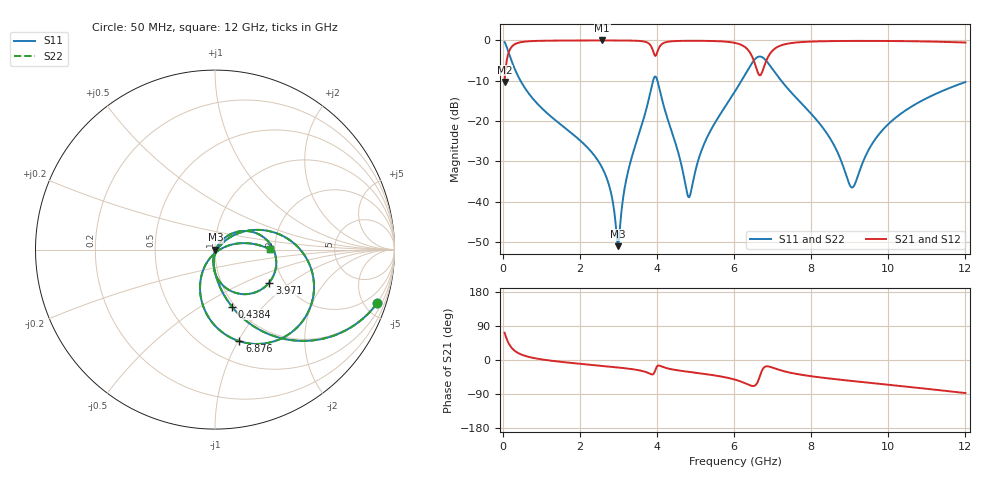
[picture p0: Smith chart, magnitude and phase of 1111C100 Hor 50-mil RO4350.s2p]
# GHz S MA R 50
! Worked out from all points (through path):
!   1601 points, 50 MHz to 12 GHz, reference 50 ohm
!   highest |S21| = -0.02 dB at 2.582 GHz (marker M1); lowest = -10.3 dB at 50 MHz (marker M2)
!   group delay of S21, straight-line fit = 21 ps
!   lowest |S11| = -51.0 dB at 2.993 GHz (marker M3), VSWR 1.01, Z = 50.3 - j0.103 ohm
!   |S11| at or under -10 dB: 462 MHz to 3.9 GHz (3.438 GHz wide, 158 % of centre); 4.013 GHz to 6.192 GHz (2.179 GHz wide, 42.7 % of centre); 7.224 GHz to end of sweep
!   |S22| runs from -51.0 to -0.4 dB; largest |S21 - S12| = 0
!   S11 on the Smith chart (normalised r, x): 50 MHz: 0.97, -6.11; 438.4 MHz: 0.97, -0.69; 3.971 GHz: 1.68, -0.70; 6.876 GHz: 0.72, -1.01; 12 GHz: 1.88, +0.01
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0.05  0.9519 -18.2  0.3062 71.8  0.3062 71.8  0.9519 -18.2
0.2367188  0.5478 -58.3  0.8361 31.6  0.8361 31.6  0.5478 -58.3
0.438375  0.3317 -73.5  0.9428 16.4  0.9428 16.4  0.3317 -73.5
2.044156  0.05549 -99.0  0.997 -10.4  0.997 -10.4  0.05549 -99.0
2.581906  0.0263 -101.7  0.9977 -15.6  0.9977 -15.6  0.0263 -101.7
2.7985  0.01359 -98.4  0.9975 -17.7  0.9975 -17.7  0.01359 -98.4
2.992688  0.002821 -21.3  0.997 -19.7  0.997 -19.7  0.002821 -21.3
3.261563  0.02492 56.0  0.9947 -22.9  0.9947 -22.9  0.02492 56.0
3.806781  0.2036 30.6  0.9004 -35.7  0.9004 -35.7  0.2036 30.6
3.971094  0.3536 -31.2  0.6485 -23.1  0.6485 -23.1  0.3536 -31.2
4.038312  0.2853 -60.0  0.7784 -14.7  0.7784 -14.7  0.2853 -60.0
4.83  0.01139 -27.6  0.9884 -31.4  0.9884 -31.4  0.01139 -27.6
5.255719  0.05639 40.8  0.9863 -37.1  0.9863 -37.1  0.05639 40.8
6.025  0.2339 27.7  0.9301 -51.8  0.9301 -51.8  0.2339 27.7
6.555281  0.5922 -21.3  0.4895 -66.4  0.4895 -66.4  0.5922 -21.3
6.68225  0.6299 -44.4  0.3708 -38.9  0.3708 -38.9  0.6299 -44.4
6.876437  0.5284 -75.1  0.6156 -16.7  0.6156 -16.7  0.5284 -75.1
7.212531  0.3215 -101.8  0.8647 -27.3  0.8647 -27.3  0.3215 -101.8
8.019156  0.1204 -120.8  0.967 -43.1  0.967 -43.1  0.1204 -120.8
9.057313  0.01503 -54.4  0.9845 -55.3  0.9845 -55.3  0.01503 -54.4
10.01331  0.09291 16.8  0.9827 -65.5  0.9827 -65.5  0.09291 16.8
12  0.3045 0.5  0.9402 -87.2  0.9402 -87.2  0.3045 0.5
